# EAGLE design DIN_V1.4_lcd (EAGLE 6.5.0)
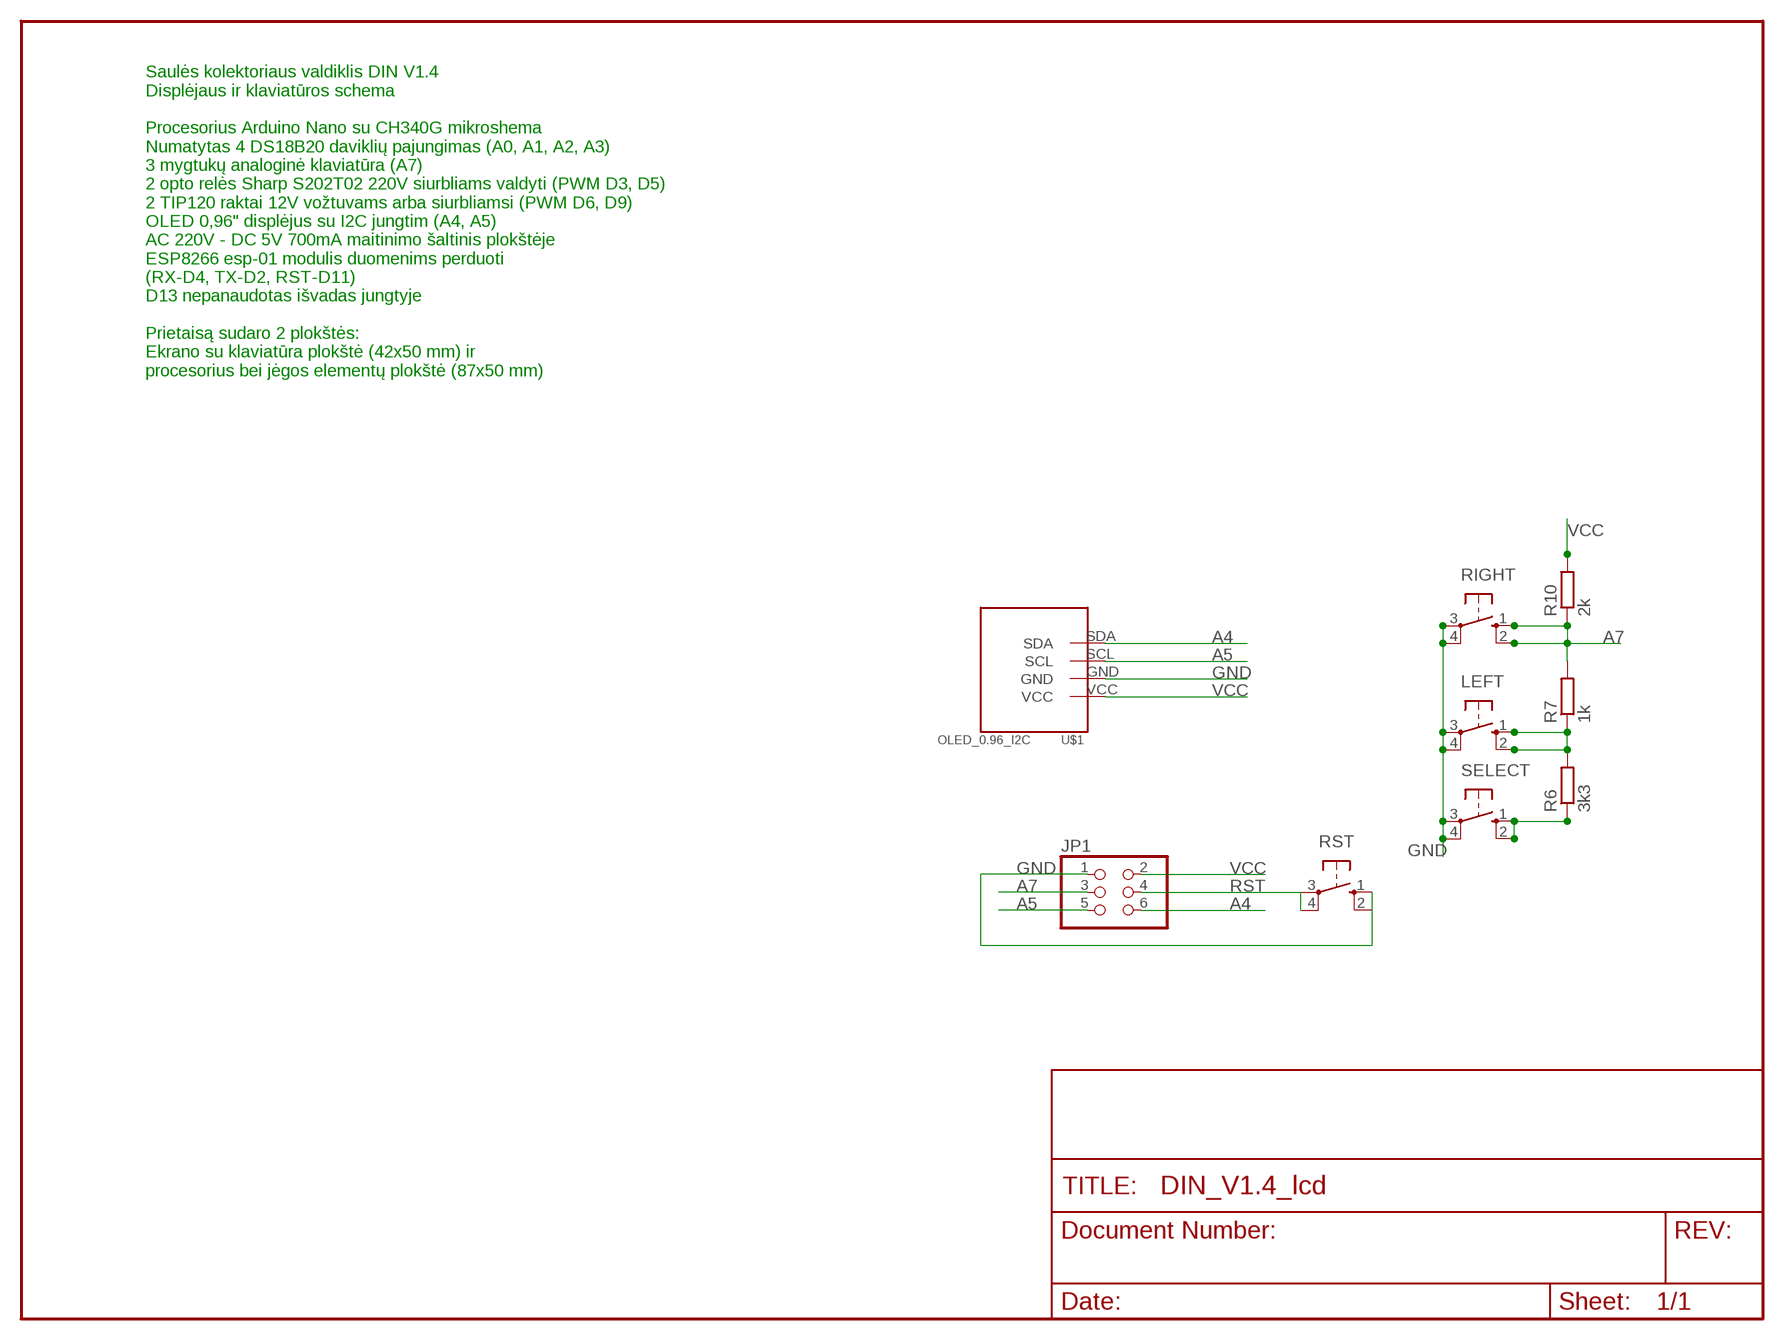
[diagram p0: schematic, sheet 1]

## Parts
JP1  PINHD-2X3  [2X03]
LEFT  10-XX  [B3F-10XX]
R6  3k3  R-EU_0207/10  [0207/10]
R7  1k  R-EU_0207/10  [0207/10]
R10  2k  R-EU_0207/10  [0207/10]
RIGHT  10-XX  [B3F-10XX]
RST  10-XX  [B3F-10XX]
SELECT  10-XX  [B3F-10XX]
U$1  OLED_0.96_I2C  [OLED_0.96_I2C]

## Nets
A4: JP1.6 U$1.SDA
A5: JP1.5 U$1.SCL
A7: JP1.3 R7.2 R10.1 RIGHT.1(S) RIGHT.2(S1)
GND [vcc]: JP1.1 LEFT.3(P) LEFT.4(P1) RIGHT.3(P) RIGHT.4(P1) RST.1(S) RST.2(S1) SELECT.3(P) SELECT.4(P1) U$1.GND
N$5: R6.1 SELECT.1(S) SELECT.2(S1)
N$6: LEFT.1(S) LEFT.2(S1) R6.2 R7.1
RST: JP1.4 RST.3(P) RST.4(P1)
VCC: JP1.2 R10.2 U$1.VCC

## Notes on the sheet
- Saulės kolektoriaus valdiklis DIN V1.4 
  Displėjaus ir klaviatūros schema
  
  Procesorius Arduino Nano su CH340G mikroshema
  Numatytas 4 DS18B20 daviklių pajungimas (A0, A1, A2, A3)
  3 mygtukų analoginė klaviatūra (A7)
  2 opto relės Sharp S202T02 220V siurbliams valdyti (PWM D3, D5)
  2 TIP120 raktai 12V vožtuvams arba siurbliamsi (PWM D6, D9)
  OLED 0,96" displėjus su I2C jungtim (A4, A5)
  AC 220V - DC 5V 700mA maitinimo šaltinis plokštėje
  ESP8266 esp-01 modulis duomenims perduoti
  (RX-D4, TX-D2, RST-D11)
  D13 nepanaudotas išvadas jungtyje
  
  Prietaisą sudaro 2 plokštės:
  Ekrano su klaviatūra plokštė (42x50 mm) ir 
  procesorius bei jėgos elementų plokštė (87x50 mm)

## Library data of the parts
JP1 = pinhead:PINHD-2X3: PIN HEADER
LEFT RIGHT RST SELECT = switch-omron:10-XX: OMRON SWITCH; MPN: B3F-1000; OC_FARNELL: 176432; OC_NEWARK: 36M3542
R6 R7 R10 = resistor:R-EU_: RESISTOR, European symbol
U$1 = tft_1.8 - Copy:OLED_0.96_I2C

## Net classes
0 default: width 0.813 mm
1 vcc: width 0.4 mm

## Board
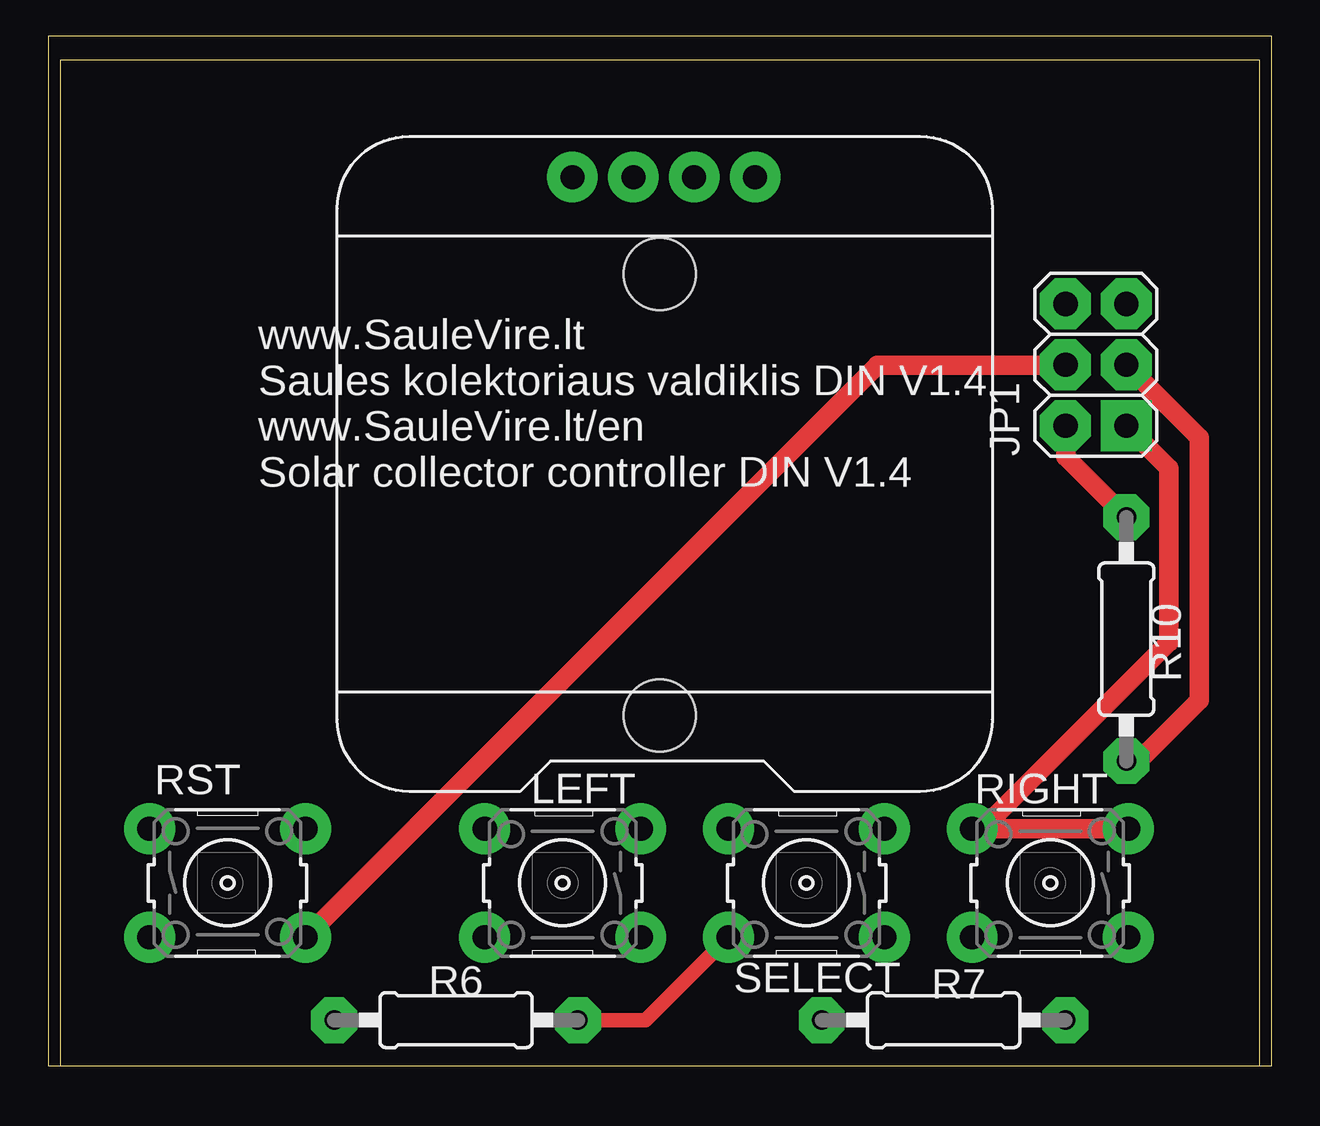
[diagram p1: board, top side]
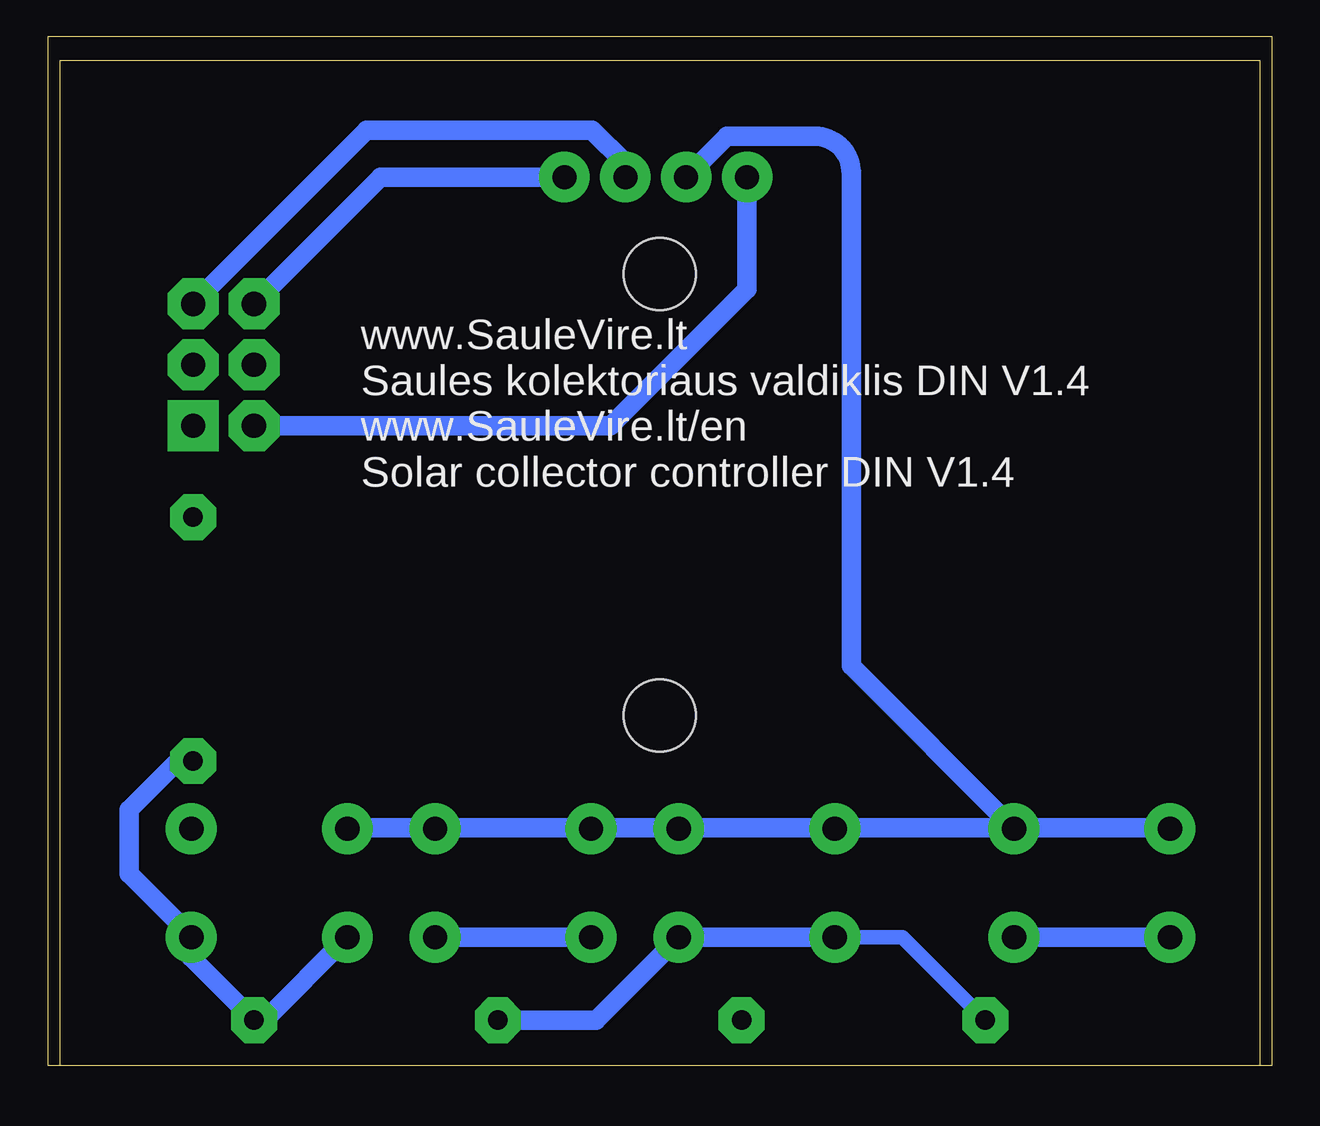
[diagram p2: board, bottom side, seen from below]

Size 50 x 41.91 mm. Coordinates in mm from the lower left corner, seen from the top.
Outline: 0,41.91 0,0 50,0 50,41.91 0,41.91
Copper layers (1*16): Top 0.035mm / dielectric 1.5mm / Bottom 0.035mm
Design rules "ITEADstudio_DRC *": minimum track width 6mil, minimum drill 12mil, track to track 6mil, track to pad 6mil, pad to pad 6mil, via to via 6mil, smd to smd 0mil, copper to edge 10mil, drill to drill 10mil, minimum pad ring 0.55mm, minimum via ring 6mil, stop-mask expansion 2mil, vias tented up to drill 100mil, thermal gap 10mil
Holes 3 mm at 25,33 25,14.61
Milling: 4 lines

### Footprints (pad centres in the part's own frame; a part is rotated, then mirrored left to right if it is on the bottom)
2X03 = drill 1.016 square: 1 -2.54,-1.27 | drill 1.016 octagon: 2 -2.54,1.27; 3 0,-1.27; 4 0,1.27; 5 2.54,-1.27; 6 2.54,1.27
B3F-10XX = drill 1.016: 1 -3.251,2.261; 2 3.251,2.261; 3 -3.251,-2.261; 4 3.251,-2.261
0207/10 = drill 0.813 octagon: 1 -5.08,0; 2 5.08,0
OLED_0.96_I2C = drill 1 pad 1.778: GND -1.63,11.63; SCL 0.91,11.63; SDA 3.45,11.63; VCC -4.17,11.63

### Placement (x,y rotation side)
JP1  43.18,29.21 90 top
LEFT  20.95,7.62 180 top
R6  16.51,1.91 180 top
R7  36.83,1.91 0 top
R10  44.45,17.78 90 top
RIGHT  41.27,7.62 180 top
RST  6.99,7.62 0 top
SELECT  31.11,7.62 180 top
U$1  25.53,25.4 0 top

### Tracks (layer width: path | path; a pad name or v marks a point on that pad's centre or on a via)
A4
  Bottom 0.813: JP1.6 36.63,37.03 U$1.SDA
A5
  Bottom 0.813: JP1.5 37.21,38.99 27.81,38.99 26.44,37.61 U$1.SCL
A7  (via drill 0.6)
  Top 0.813: JP1.3 47.5,26.16 47.5,15.24 44.96,12.7 R10.1
  Bottom 0.42: 44.48,12.7 44.48,12.64 R10.1 | 44.64,5.52 RIGHT.1 | v44.48,29.36 44.48,29.2 JP1.3
  Bottom 0.813: 44.64,5.52 47.12,8 47.12,10.67 45.09,12.7 R10.1 | RIGHT.2 41.48,1.91 R7.2 44.53,4.52 RIGHT.1
GND
  Top 0.813: RIGHT.3 RIGHT.4 38.46,9.88 46.23,17.65 46.23,24.89 JP1.1
  Bottom 0.4: 3.81,9.92 3.76,9.92 RST.1 | 10.16,9.92 RST.2 10.4,9.92 | 17.76,9.92 LEFT.4 17.52,9.92 | 24.16,9.92 LEFT.3 24.4,9.92 | 27.84,9.92 SELECT.4 28,9.92 | 34.4,9.92 SELECT.3 34.24,9.92 | 38,9.92 RIGHT.4
  Bottom 0.813: 10.16,9.92 3.81,9.92 | 24.16,9.92 17.76,9.92 | 24.4,9.92 27.84,9.92 | 17.52,9.92 10.4,9.92 | 38,9.92 34.4,9.92 | 34.24,9.92 28,9.92 | RST.2 17.02,16.66 17.02,23.11 17.02,37.21 arc-90 18.54,38.73 20.16,38.73 22.19,38.73 U$1.GND
N$5
  Top 0.61: SELECT.2 24.41,1.91 R6.1
  Bottom 0.42: 27.92,5.36 SELECT.2 | 34.16,5.36 SELECT.1
  Bottom 0.813: 34.16,5.36 27.92,5.36
N$6
  Bottom 0.42: 17.92,5.36 LEFT.2 | 24,5.36 LEFT.1
  Bottom 0.61: LEFT.2 14.88,5.36 R6.2
  Bottom 0.813: 24,5.36 17.92,5.36 | R7.1 27.66,1.91 LEFT.1
RST
  Top 0.42: 41.84,29.2 JP1.4 | RST.4
  Top 0.813: 41.84,29.2 34.08,29.2 RST.4
  Bottom 0.42: 3.76,5.36 RST.3 | 10.16,5.36 RST.4
  Bottom 0.813: 10.16,5.36 3.76,5.36
VCC  (via drill 0.6)
  Top 0.813: v44.4,22.89 41.92,25.37 JP1.2
  Bottom 0.42: v44.4,22.89 v44.4,22.88 R10.2
  Bottom 0.813: JP1.2 29.68,26.67 27.05,26.67 21.36,32.36 U$1.VCC

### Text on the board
tPlace: www.SauleVire.lt / Saules kolektoriaus valdiklis DIN V1.4 / www.SauleVire.lt/en / Solar collector controller DIN V1.4
bPlace: www.SauleVire.lt / Saules kolektoriaus valdiklis DIN V1.4 / www.SauleVire.lt/en / Solar collector controller DIN V1.4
